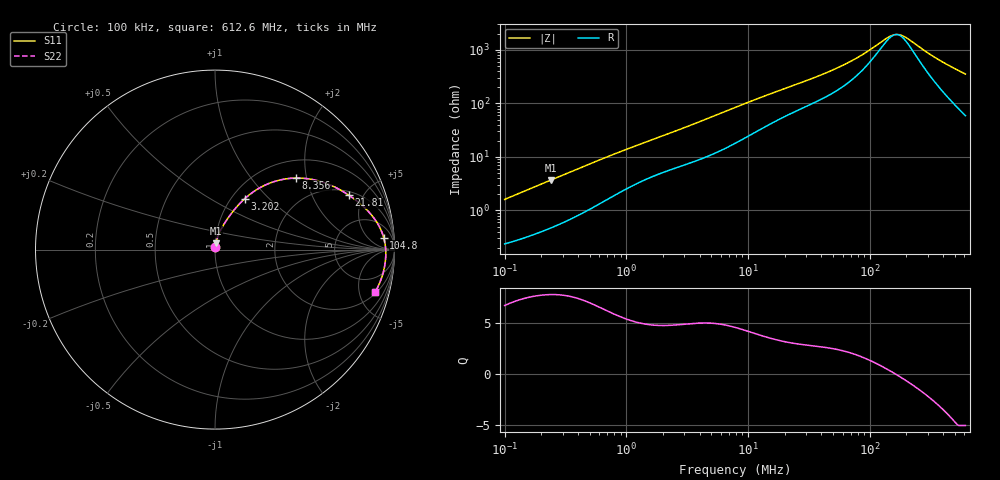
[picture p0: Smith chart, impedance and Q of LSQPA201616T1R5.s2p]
! LSQPA201616T1R5  S-PARAMETER MODEL  ( General Type )
! Model Generated by TAIYO YUDEN Corporation (http://www.ty-top.com)
! Version 2.0
! TAIYO YUDEN Control No. 100810NF25SB-FKC
! Copyright(c) 2007 TAIYO YUDEN CO.,LTD. All Rights Reserved.
! Product Description (link to TY-COMPAS)
! https://ds.yuden.co.jp/TYCOMPAS/or/detail?pn=LSQPA201616T1R5M&u=M
! Products Name : Inductors
! Characteristics :
!  Inductance : 1.5 uH , SRF(min) : 80 MHz , DC Resistance(max) : 0.195 Ohm
!  Rated Current : Saturation :1000 mA , Temp Rise : 1000 mA (40 degC)
!  Case Size : 2.0 x 1.6 / 0.079 x 0.063 [mm/inch] , Thickness : 1.6 / 0.063 [mm/inch]
!  (Conditions: Temperature = 25 degC , DC Bias Current/Voltage = 0A / 0V)
! External Node Assignments :
!  1  o---GGG---o  2
! GND o---------o GND
! Frequency Range : 0.1MHz  -  612.621916MHz  [ 402 STEP ]
# MHz S RI R 50
! Freq[MHz].  S11 Real  S11 Imag  S21 Real  S21 Imag  S12 Real  S12 Imag  S22 Real  S22 Imag
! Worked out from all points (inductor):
!   401 points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, 100 kHz to 612.6 MHz, reference 50 ohm
!   read as one part in series: L = 2.5 uH near 104.5 kHz
!   highest Q = 7.78 at 239.2 kHz (marker M1), where L = 2.43 uH
!   self-resonance near 164.5 MHz
!   S11 on the Smith chart (normalised r, x): 100 kHz: 1.00, +0.03; 3.202 MHz: 1.15, +0.73; 8.356 MHz: 1.39, +1.74; 21.81 MHz: 2.25, +3.86; 104.8 MHz: 14, +17; 612.6 MHz: 2.18, -6.99
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0.1  0.00261 0.0158  0.9974 -0.0158  0.9974 -0.0158  0.00261 0.0158
0.239177  0.00598 0.0361  0.994 -0.0361  0.994 -0.0361  0.00598 0.0361
0.430878  0.0126 0.0623  0.9874 -0.0623  0.9874 -0.0623  0.0126 0.0623
0.9445  0.0383 0.1216  0.9617 -0.1216  0.9617 -0.1216  0.0383 0.1216
1.856562  0.0891 0.1988  0.9109 -0.1988  0.9109 -0.1988  0.0891 0.1988
3.201909  0.1656 0.2838  0.8344 -0.2838  0.8344 -0.2838  0.1656 0.2838
4.845077  0.265 0.3525  0.735 -0.3525  0.735 -0.3525  0.265 0.3525
7.827017  0.4281 0.3976  0.5719 -0.3976  0.5719 -0.3976  0.4281 0.3976
8.356034  0.4523 0.3987  0.5477 -0.3987  0.5477 -0.3987  0.4523 0.3987
13.79634  0.6259 0.3665  0.3741 -0.3665  0.3741 -0.3665  0.6259 0.3665
21.80677  0.7449 0.3035  0.2551 -0.3035  0.2551 -0.3035  0.7449 0.3035
33.72493  0.8277 0.2385  0.1723 -0.2385  0.1723 -0.2385  0.8277 0.2385
46.77036  0.8753 0.1885  0.1247 -0.1885  0.1247 -0.1885  0.8753 0.1885
63.46327  0.9084 0.1411  0.0916 -0.1411  0.0916 -0.1411  0.9084 0.1411
82.44005  0.9283 0.1009  0.0717 -0.1009  0.0717 -0.1009  0.9283 0.1009
104.7818  0.9404 0.0651  0.0596 -0.0651  0.0596 -0.0651  0.9404 0.0651
145.3134  0.9495 0.0178  0.0505 -0.0178  0.0505 -0.0178  0.9495 0.0178
165.6203  0.9511 -0.000985  0.0489 0.000985  0.0489 0.000985  0.9511 -0.000985
188.765  0.9517 -0.02  0.0483 0.02  0.0483 0.02  0.9517 -0.02
355.2164  0.9386 -0.1222  0.0614 0.1222  0.0614 0.1222  0.9386 -0.1222
481.9974  0.9186 -0.1828  0.0814 0.1828  0.0814 0.1828  0.9186 -0.1828
612.6219  0.8921 -0.2371  0.1079 0.2371  0.1079 0.2371  0.8921 -0.2371
